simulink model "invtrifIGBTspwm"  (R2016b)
settings: Solver=VariableStepAuto  StartTime=0.0  StopTime=5  RelTol=1e-3
undefined symbols (not defined in the file): bridge, phase, pulses, Three
libraries: powerlib x17, powerlib_meascontrol x4

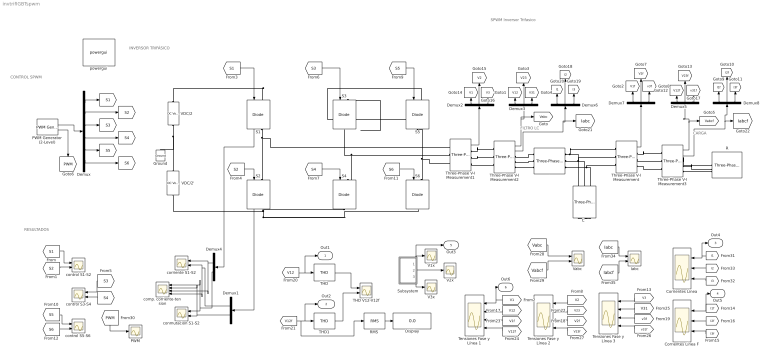
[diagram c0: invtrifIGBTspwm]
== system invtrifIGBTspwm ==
  note: RESULTADOS
  note: CONTROL SPWM
  note: INVERSOR TRIFÁSICO
  note: CARGA
  note: FILTRO LC
  note: SPWM Inversor Trifasico
  "C  " : powerlib/Elements/Three-Phase Series RLC Branch  LConnTagsString=A|B|C  RConnTagsString=A|B|C  BranchType=C  Resistance=1  Inductance=1e-3  Capacitance=1e-4  Measurements=None
  Corrientes Línea : Scope  NumInputPorts=3
  Corrientes Línea F : Scope  NumInputPorts=3
  Demux : Demux  Outputs=6
  Demux1 : Demux  Outputs=2
  Demux{2..3,5..8} (6 alike) : Demux  Outputs=3
  Demux4 : Demux  Outputs=2
  Display : Display
  Ground : powerlib/Elements/Ground  LConnTagsString=a
  Iabc : Scope  NumInputPorts=2
  L : powerlib/Elements/Three-Phase Series RLC Branch  LConnTagsString=A|B|C  RConnTagsString=A|B|C  BranchType=L  Resistance=40  Inductance=10e-3  Capacitance=1e-6  Measurements=Branch voltages and currents
  PWM : Scope
  PWM Generator (2-Level) : powerlib_meascontrol/Pulse & Signal Generators/PWM Generator (2-Level)  ModulatorType=Three-phase bridge (6 pulses)  ModulatorMode=Unsynchronized  Fc=1050  Pc=90  nF=27  MinMax="[ -1  1 ]"  SamplingTechnique=Natural  ModulatingSignals=on  m=0.85  Freq=50  Phase=0  Ts=0  ShowCarrierOutport=on
  R : powerlib/Elements/Three-Phase Series RLC Load  LConnTagsString=A|B|C  Configuration=Y (grounded)  NominalVoltage=220  Vabc=[1e3 1e3 1e3]  Vabcp=[1e3 1e3 1e3]  NominalFrequency=50  UnbalancedPower=off  ActivePower=2430  InductivePower=1177  CapacitivePower=0  Pabc=[10e3 9e3 11e3]  QLabc=[100 90 110]  QCabc=[100 90 110]  Pabcp=[10e3 9e3 11e3]  QLabcp=[100 90 110]  QCabcp=[100 90 110]  Measurements=None  LoadType=constant Z
  "RMS " : powerlib_meascontrol/Measurements/RMS  TrueRMS=on  Freq=50  RMSInit=220  Ts=0
  S1 : powerlib/Power Electronics/IGBT//Diode  Ron=1e-3  Rs=1e5  Cs=inf  Measurements=on
  S2 : powerlib/Power Electronics/IGBT//Diode  Ron=1e-3  Rs=1e5  Cs=inf  Measurements=on
  S{3..6} (4 alike) : powerlib/Power Electronics/IGBT//Diode  Ron=1e-3  Rs=1e5  Cs=inf  Measurements=off
  Subsystem : Subsystem
  THD : powerlib_meascontrol/Measurements/THD  Freq=50  Ts=0
  THD V12-V12f : Scope  NumInputPorts=2
  THD1 : powerlib_meascontrol/Measurements/THD  Freq=50  Ts=0
  Tensiones Fase y Línea 1 : Scope  NumInputPorts=4
  Tensiones Fase y Línea 2 : Scope  NumInputPorts=4
  Tensiones Fase y Línea 3 : Scope  NumInputPorts=4
  Three-Phase V-I Measurement : powerlib/Measurements/Three-Phase V-I Measurement  VoltageMeasurement=phase-to-ground  SetLabelV=off  LabelV=Vabc  Vpu=off  VpuLL=off  CurrentMeasurement=no  SetLabelI=off  LabelI=Iabc  Ipu=off  Pbase=100e6  Vbase=500e3  OutputType=Complex  PhasorSimulation=off  PSBequivalent=0
  Three-Phase V-I Measurement1 : powerlib/Measurements/Three-Phase V-I Measurement  VoltageMeasurement=phase-to-ground  SetLabelV=off  LabelV=Vabc  Vpu=off  VpuLL=off  CurrentMeasurement=no  SetLabelI=off  LabelI=Iabc  Ipu=off  Pbase=100e6  Vbase=500e3  OutputType=Complex  PhasorSimulation=off  PSBequivalent=0
  Three-Phase V-I Measurement2 : powerlib/Measurements/Three-Phase V-I Measurement  VoltageMeasurement=phase-to-phase  SetLabelV=off  LabelV=Vabc  Vpu=off  VpuLL=off  CurrentMeasurement=yes  SetLabelI=off  LabelI=Iabc  Ipu=off  Pbase=100e6  Vbase=500e3  OutputType=Complex  PhasorSimulation=off  PSBequivalent=0
  Three-Phase V-I Measurement3 : powerlib/Measurements/Three-Phase V-I Measurement  VoltageMeasurement=phase-to-phase  SetLabelV=off  LabelV=Vabc  Vpu=off  VpuLL=off  CurrentMeasurement=yes  SetLabelI=off  LabelI=Iabc  Ipu=off  Pbase=100e6  Vbase=500e3  OutputType=Complex  PhasorSimulation=off  PSBequivalent=0
  V1x : Scope
  V2x : Scope
  V3x : Scope
  VDC/2 : powerlib/Electrical Sources/DC Voltage Source  Amplitude=210  Measurements=None
  VDC/2' : powerlib/Electrical Sources/DC Voltage Source  Amplitude=210  Measurements=None
  "Vabc " : Scope  NumInputPorts=2
  comp. corriente-tension : Scope  NumInputPorts=4
  conmutacion S1-S2 : Scope  NumInputPorts=2
  control S1-S2 : Scope  NumInputPorts=2
  control S3-S4 : Scope  NumInputPorts=2
  "control S5-S6 " : Scope  NumInputPorts=2
  corriente S1-S2 : Scope  NumInputPorts=2
  powergui : powerlib/powergui  Priority=1  SimulationMode=Continuous  SolverType=Tustin/Backward Euler (TBE)  SampleTime=5e-5  frequency=60  SPID=off  DisableSnubberDevices=off  DisableRonSwitches=off  DisableVfSwitches=off  SwTol=0  DisplayEquations=off  Interpol=off  ExternalGateDelay=off  methode=off  Ts=10  FunctionMessages=off  echomessages=off  HookPort=off  EnableUseOfTLC=off  x0status=blocks  frequencyindice=0  Pbase=100e6  ErrMax=1e-4  Iterations=50  UnitsV=kV  UnitsW=MW  buscounter=0  RestoreLinks=warning  ResistiveCurrentMeasurement=off  Frange=[0:2:500]  Ylog=off  Xlog=on  ShowGrid=off  save=off  variable=ZData  structure=yout  ZoomFFT=off  StartTime=0.0389  cycles=1  DisplayStyle=2  fundamental=50  FreqAxis=off  MaxFrequency=7800  frequencyindicesteady=1  RmsSteady=1  display=off
  Out1 : Outport  SignalName=V12
  Out2 : Outport  Port=2  SignalName=V12f
  Out4 : Outport  Port=3  SignalName=I1
  Out5 : Outport  Port=4  SignalName=I1f
  Out3 : Outport  Port=5  SignalName=V1x
  Out6 : Outport  Port=6  SignalName=V1
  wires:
  PWM Generator (2-Level)/1 -> Demux/1
  [S1] -> S1/1
  [S2] -> S2/1
  [S3] -> S3/1
  [S4] -> S4/1
  [S6] -> S6/1
  [S5] -> S5/1
  S2/1 -> Demux1/1
  S1/1 -> Demux4/1
  [S1] -> control S1-S2/1
  [S2] -> control S1-S2/2
  [S3] -> control S3-S4/1
  [S4] -> control S3-S4/2
  [S5] -> "control S5-S6 "/1
  [S6] -> "control S5-S6 "/2
  Demux/2 -> [S2]
  Demux/1 -> [S1]
  Demux/3 -> [S3]
  Demux/4 -> [S4]
  Demux/5 -> [S5]
  Demux/6 -> [S6]
  Three-Phase V-I Measurement/1 -> Demux7/1
  Demux7/1 -> [V1f]
  Demux7/2 -> [V2f]
  Demux7/3 -> [v3f]
  [V1] -> Out6/1, Tensiones Fase y Línea 1/1
  [V2] -> Tensiones Fase y Línea 2/1
  Demux8/2 -> [I2f]
  Demux8/1 -> [I1f]
  Demux8/3 -> [I3f]
  Demux1/1 -> comp. corriente-tension/4, corriente S1-S2/2
  Demux4/1 -> comp. corriente-tension/3, corriente S1-S2/1
  Demux4/2 -> comp. corriente-tension/1, conmutacion S1-S2/1
  Demux1/2 -> comp. corriente-tension/2, conmutacion S1-S2/2
  Three-Phase V-I Measurement1/1 -> Demux2/1
  Demux2/2 -> [V2]
  Demux2/3 -> [V3]
  [V2f] -> Tensiones Fase y Línea 2/3
  [V23] -> Tensiones Fase y Línea 2/2
  [I2f] -> Corrientes Línea F/2
  [I1f] -> Out5/1, Corrientes Línea F/1
  [I3f] -> Corrientes Línea F/3
  Three-Phase V-I Measurement2/1 -> Demux3/1, [Vabc]
  Demux3/1 -> [V12]
  Demux3/2 -> [V23]
  Demux3/3 -> [V31]
  [V12] -> Tensiones Fase y Línea 1/2
  Three-Phase V-I Measurement3/1 -> Demux5/1, [Vabcf]
  Demux5/1 -> [V12f]
  Demux5/2 -> [V23f]
  Demux5/3 -> [v31f]
  [V3] -> Tensiones Fase y Línea 3/1
  [v3f] -> Tensiones Fase y Línea 3/3
  [V1f] -> Tensiones Fase y Línea 1/3
  [V12f] -> Tensiones Fase y Línea 1/4
  [V31] -> Tensiones Fase y Línea 3/2
  [v31f] -> Tensiones Fase y Línea 3/4
  [V23f] -> Tensiones Fase y Línea 2/4
  THD/1 -> THD V12-V12f/1
  [V12] -> Out1/1, THD/1
  THD1/1 -> THD V12-V12f/2
  [Vabc] -> "Vabc "/1
  [Vabcf] -> "Vabc "/2
  PWM Generator (2-Level)/2 -> [PWM]
  [PWM] -> PWM/1
  [V12f] -> "RMS "/1, Out2/1, THD1/1
  "RMS "/1 -> Display/1
  Three-Phase V-I Measurement3/2 -> Demux8/1, [Iabcf]
  Demux2/1 -> [V1]
  Three-Phase V-I Measurement2/2 -> [Iabc], Demux6/1
  Demux6/2 -> [I2]
  Demux6/1 -> [I1]
  Demux6/3 -> [I3]
  [I2] -> Corrientes Línea/2
  [I1] -> Out4/1, Corrientes Línea/1
  [I3] -> Corrientes Línea/3
  [Iabc] -> Iabc/1
  [Iabcf] -> Iabc/2
  Subsystem/2(Out2) -> V2x/1
  Subsystem/3(Out3) -> V3x/1
  Subsystem/1(Out1) -> Out3/1, V1x/1
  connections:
  VDC/2'/LConn1 -- S6/RConn1 -- S4/RConn1 -- S2/RConn1
  VDC/2/RConn1 -- S1/LConn1 -- S5/LConn1 -- S3/LConn1
  S5/RConn1 -- Three-Phase V-I Measurement1/LConn3 -- S6/LConn1
  VDC/2/LConn1 -- Ground/LConn1 -- VDC/2'/RConn1
  L/RConn1 -- "C  "/LConn1 -- Three-Phase V-I Measurement/LConn1
  L/RConn2 -- "C  "/LConn2 -- Three-Phase V-I Measurement/LConn2
  L/RConn3 -- "C  "/LConn3 -- Three-Phase V-I Measurement/LConn3
  S1/RConn1 -- Three-Phase V-I Measurement1/LConn1 -- S2/LConn1
  "C  "/RConn1 -- "C  "/RConn3 -- "C  "/RConn2
  L/LConn1 -- Three-Phase V-I Measurement2/RConn1
  L/LConn2 -- Three-Phase V-I Measurement2/RConn2
  L/LConn3 -- Three-Phase V-I Measurement2/RConn3
  Three-Phase V-I Measurement1/RConn1 -- Three-Phase V-I Measurement2/LConn1
  Three-Phase V-I Measurement1/RConn2 -- Three-Phase V-I Measurement2/LConn2
  Three-Phase V-I Measurement1/RConn3 -- Three-Phase V-I Measurement2/LConn3
  Three-Phase V-I Measurement/RConn1 -- Three-Phase V-I Measurement3/LConn1
  Three-Phase V-I Measurement/RConn2 -- Three-Phase V-I Measurement3/LConn2
  Three-Phase V-I Measurement/RConn3 -- Three-Phase V-I Measurement3/LConn3
  Three-Phase V-I Measurement3/RConn1 -- R/LConn1
  Three-Phase V-I Measurement3/RConn2 -- R/LConn2
  Three-Phase V-I Measurement3/RConn3 -- R/LConn3
  Three-Phase V-I Measurement1/LConn2 -- S3/RConn1 -- S4/LConn1

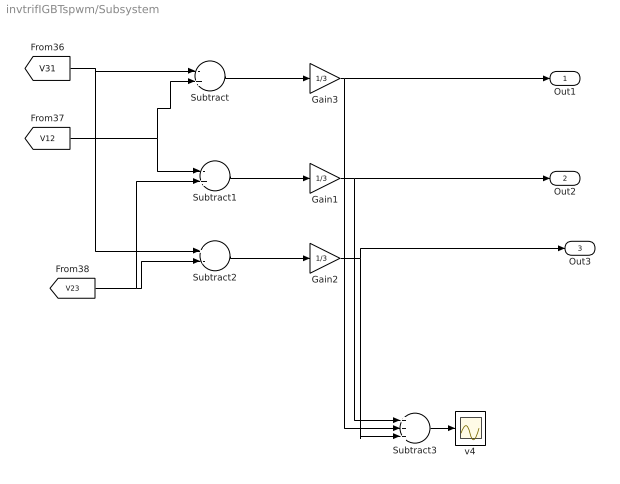
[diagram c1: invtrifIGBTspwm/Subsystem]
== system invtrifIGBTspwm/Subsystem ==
  Gain1 : Gain  Gain=1/3
  Gain2 : Gain  Gain=1/3
  Gain3 : Gain  Gain=1/3
  Subtract : Sum  Inputs=-+
  Subtract1 : Sum  Inputs=-+
  Subtract2 : Sum  Inputs=+-
  Subtract3 : Sum  Inputs=+++
  v4 : Scope
  Out1 : Outport
  Out2 : Outport  Port=2
  Out3 : Outport  Port=3
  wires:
  [V23] -> Subtract1/2, Subtract2/2
  Subtract3/1 -> v4/1
  [V12] -> Subtract/2, Subtract1/1
  [V31] -> Subtract2/1, Subtract/1
  Subtract2/1 -> Gain2/1
  Subtract1/1 -> Gain1/1
  Gain2/1 -> Out3/1, Subtract3/3
  Gain1/1 -> Out2/1, Subtract3/1
  Gain3/1 -> Out1/1, Subtract3/2
  Subtract/1 -> Gain3/1
